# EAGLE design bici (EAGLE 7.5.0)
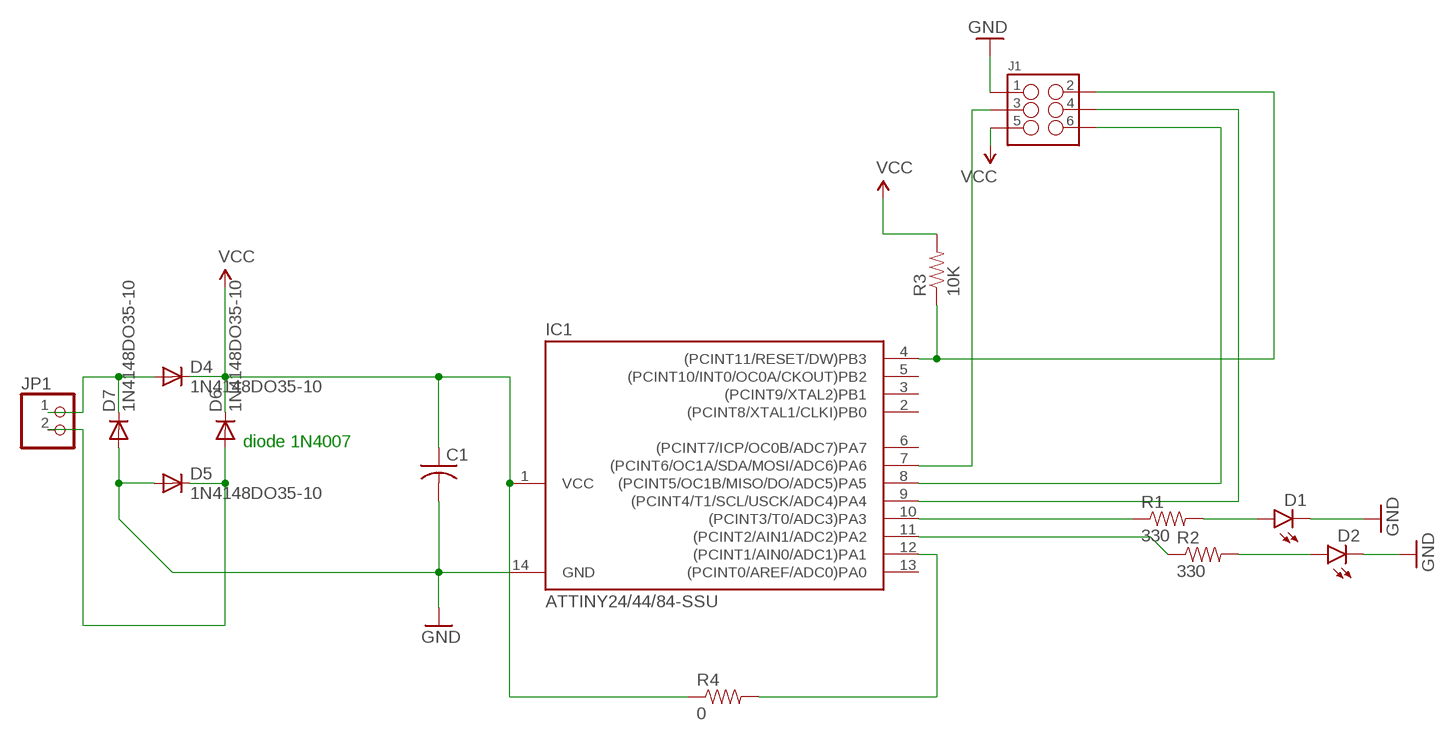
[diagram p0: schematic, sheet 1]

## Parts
C1  C-US050-050X075  [C050-050X075]
D1  LED3MM  [LED3MM]
D2  LED3MM  [LED3MM]
D4  1N4148DO35-10  [DO35-10]
D5  1N4148DO35-10  [DO35-10]
D6  1N4148DO35-10  [DO35-10]
D7  1N4148DO35-10  [DO35-10]
IC1  ATTINY24/44/84-SSU  [SOIC14]
J1  M03X2  [2X3_SMD]
JP1  PINHD-1X2  [1X02]
R1  330  RESISTOR1206  [1206]
R2  330  RESISTOR1206  [1206]
R3  10K  RESISTOR1206  [1206]
R4  0  RESISTOR1206  [1206]

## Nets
GND: C1.2 D1.K(C) D2.K(C) D5.A D7.A J1.1
MISO: IC1.8((PCINT5/OC1B/MISO/DO/ADC5)PA5) J1.6
MOSI: IC1.7((PCINT6/OC1A/SDA/MOSI/ADC6)PA6) J1.3
N$1: IC1.10((PCINT3/T0/ADC3)PA3) R1.1
N$2: D1.A R1.2
N$3: D4.A D7.C JP1.1
N$4: IC1.12((PCINT1/AIN0/ADC1)PA1) R4.2
N$5: D5.C D6.A JP1.2
N$7: IC1.11((PCINT2/AIN1/ADC2)PA2) R2.1
N$8: D2.A R2.2
RST: IC1.4((PCINT11/RESET/DW)PB3) J1.2 R3.1
SCK: IC1.9((PCINT4/T1/SCL/USCK/ADC4)PA4) J1.4
VCC: C1.1 D4.C D6.C IC1.1(VCC) J1.5 R3.2 R4.1
Unconnected: IC1.2((PCINT8/XTAL1/CLKI)PB0) IC1.3((PCINT9/XTAL2)PB1) IC1.5((PCINT10/INT0/OC0A/CKOUT)PB2) IC1.6((PCINT7/ICP/OC0B/ADC7)PA7) IC1.13((PCINT0/AREF/ADC0)PA0)

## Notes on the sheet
- diode 1N4007

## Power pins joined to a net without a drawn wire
GND: IC1.14(GND)

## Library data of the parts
C1 = rcl:C-US: CAPACITOR, American symbol
D1 D2 = SparkFun-LED:LED: LEDs; PROD_ID: DIO-08794
D4-D7 = diode:1N4148: DIODE
IC1 = attiny24_44_84:ATTINY24/44/84
J1 = SparkFun-Connectors:M03X2: 2x3 .1" header. Shrouded, with keying- CONN-10681 SMT- CONN-11415 Pogo pins- HW-11044; PROD_ID: CONN-11290
JP1 = pinhead:PINHD-1X2: PIN HEADER
R1-R4 = SparkFun-Resistors:RESISTOR: Resistor

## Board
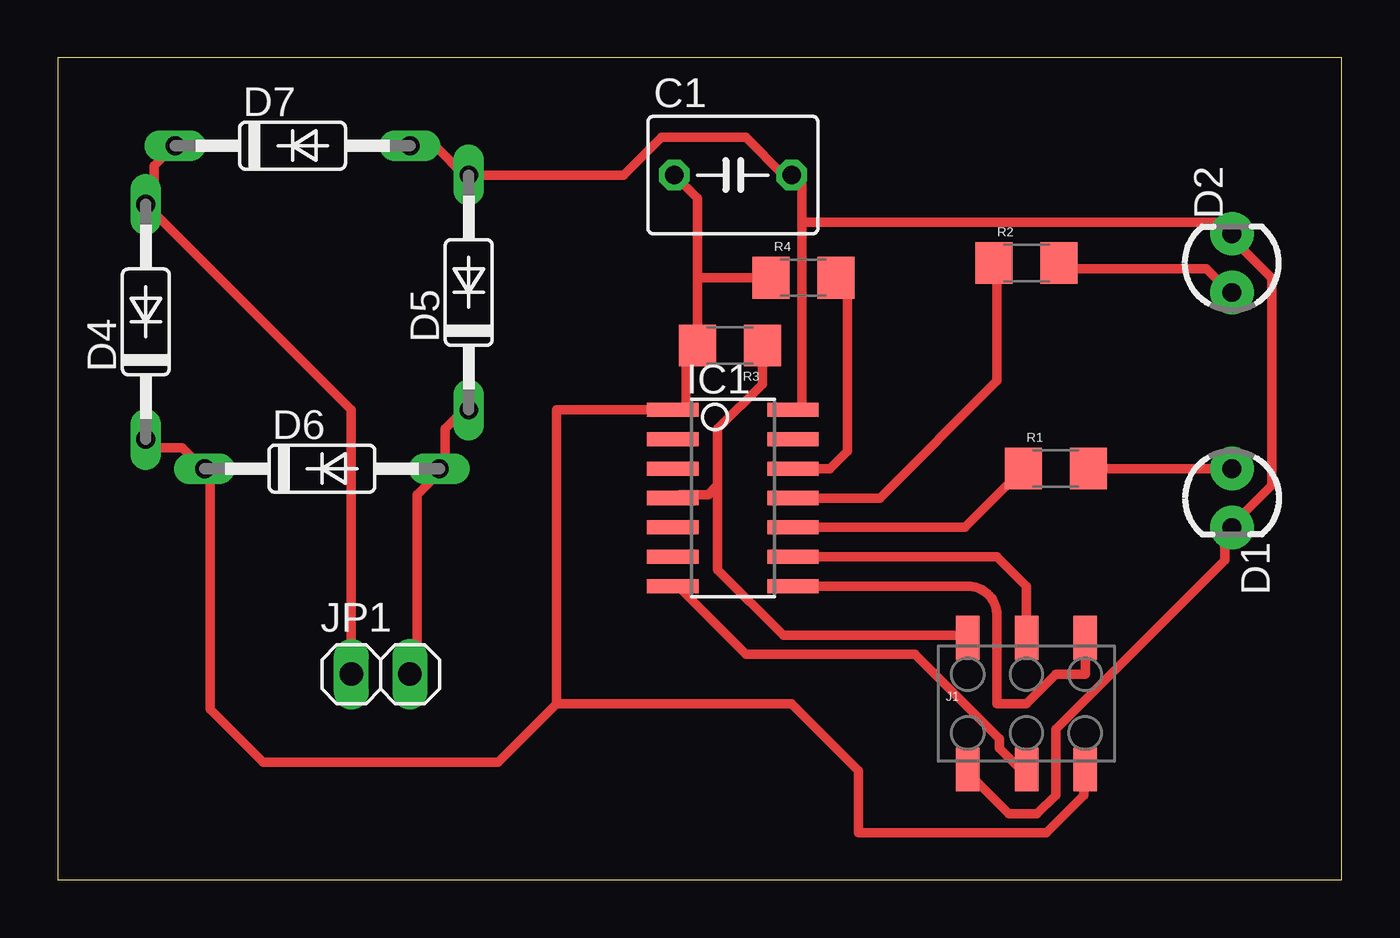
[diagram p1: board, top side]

Size 55.55 x 35.55 mm. Coordinates in mm from the lower left corner, seen from the top.
Outline: 0,35.55 0,0 55.55,0 55.55,35.55 0,35.55
Copper layers (1*16): Top 0.035mm / dielectric 1.5mm / Bottom 0.035mm
Design rules "default *": minimum track width 16mil, minimum drill 24mil, track to track 16mil, track to pad 16mil, pad to pad 16mil, via to via 16mil, smd to smd 15mil, copper to edge 40mil, drill to drill 8mil, minimum pad ring 10mil, minimum via ring 8mil, stop-mask expansion 4mil, vias tented up to drill 0mil, thermal gap 10mil

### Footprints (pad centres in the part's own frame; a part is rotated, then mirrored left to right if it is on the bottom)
C050-050X075 = drill 0.813 octagon: 1 -2.54,0; 2 2.54,0
LED3MM = drill 0.813 pad 1.88: A -1.27,0; K 1.27,0
DO35-10 = drill 0.813 long: A 5.08,0; C -5.08,0
SOIC14 = smd 0.61 x 2.21: 1 -3.81,-2.603; 2 -2.54,-2.603; 3 -1.27,-2.603; 4 0,-2.603; 5 1.27,-2.603; 6 2.54,-2.603; 7 3.81,-2.603; 8 3.81,2.603; 9 2.54,2.603; 10 1.27,2.603; 11 0,2.603; 12 -1.27,2.603; 13 -2.54,2.603; 14 -3.81,2.603
2X3_SMD = smd 1.02 x 1.9: 1 -2.54,-2.85; 2 -2.54,2.85; 3 0,-2.85; 4 0,2.85; 5 2.54,-2.85; 6 2.54,2.85
1X02 = drill 1.016 long: 1 -1.27,0; 2 1.27,0
1206 = smd 1.6 x 1.8: 1 -1.4,0; 2 1.4,0

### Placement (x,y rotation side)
C1  29.21,30.48 0 top
D1  50.8,16.51 270 top
D2  50.8,26.67 90 top
D4  3.81,24.13 90 top
D5  17.78,25.4 90 top
D6  11.43,17.78 0 top
D7  10.16,31.75 0 top
IC1  29.21,16.51 270 top
J1  41.91,7.62 0 top
JP1  13.97,8.89 0 top
R1  43.18,17.78 0 top
R2  41.91,26.67 0 top
R3  29.08,23.11 180 top
R4  32.26,26.04 0 top

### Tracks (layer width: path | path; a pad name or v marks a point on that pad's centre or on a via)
GND
  Top 0.406: D7.A 15.54,31.7 16.36,31.7 17.58,30.48 D5.A 24.49,30.48 26.11,32.11 29.77,32.11 31.39,30.48 C1.2 31.8,30.48 32.21,30.07 32.21,28.45 | 32.21,28.45 32.21,20.32 IC1.14 | J1.1 39.52,4.47 41.15,2.85 42.37,2.85 43.18,3.66 43.18,6.5 50.49,13.82 50.49,15.04 D1.K 50.9,15.44 52.53,17.07 52.53,26.01 50.9,27.64 D2.K 50.49,28.04 50.09,28.45 32.21,28.45
MISO
  Top 0.406: J1.6 44.45,8.89 43.18,8.89 41.91,7.62 40.64,7.62 40.64,11.43 arc90 39.37,12.7 IC1.8
MOSI
  Top 0.406: J1.3 41.55,4.88 40.74,5.69 40.74,6.1 37.08,9.75 29.77,9.75 26.92,12.6 IC1.7
N$1
  Top 0.406: IC1.10 39.24,15.24 R1.1
N$2
  Top 0.406: R1.2 D1.A
N$3
  Top 0.406: D7.C 4.98,31.7 4.17,30.89 4.17,29.26 D4.A 12.7,20.32 JP1.1
N$4
  Top 0.406: IC1.12 33.4,17.78 34.16,18.54 34.16,25.53 R4.2
N$5
  Top 0.406: D5.C 17.58,20.32 16.76,19.51 16.76,17.88 D6.A 16.36,17.48 15.54,16.66 15.54,8.94 JP1.2
N$7
  Top 0.406: IC1.11 35.56,16.51 40.64,21.59 40.64,26.54 R2.1
N$8
  Top 0.406: R2.2 43.59,26.42 49.68,26.42 50.49,25.6 D2.A
RST
  Top 0.406: 28.55,17.07 28.55,19.51 30.48,21.44 R3.1 | 28.55,17.07 28.14,16.66 26.92,16.66 IC1.4 | 28.55,17.07 28.55,13.41 31.39,10.57 39.12,10.57 J1.2
SCK
  Top 0.406: IC1.9 40.64,13.97 41.91,12.7 J1.4
VCC
  Top 0.406: D4.C 4.17,18.69 5.38,18.69 6.2,17.88 D6.C 6.6,17.48 6.6,7.37 8.89,5.08 19.05,5.08 21.59,7.62 | J1.5 44.4,4.47 44.4,3.66 42.77,2.03 34.65,2.03 34.65,4.72 31.75,7.62 21.59,7.62 | 21.59,7.62 21.59,20.32 IC1.1 26.92,20.32 27.18,20.57 27.18,22.99 27.3,23.11 R3.2 27.68,26.04 | C1.1 27.68,29.47 27.68,26.04 | R4.1 27.68,26.04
